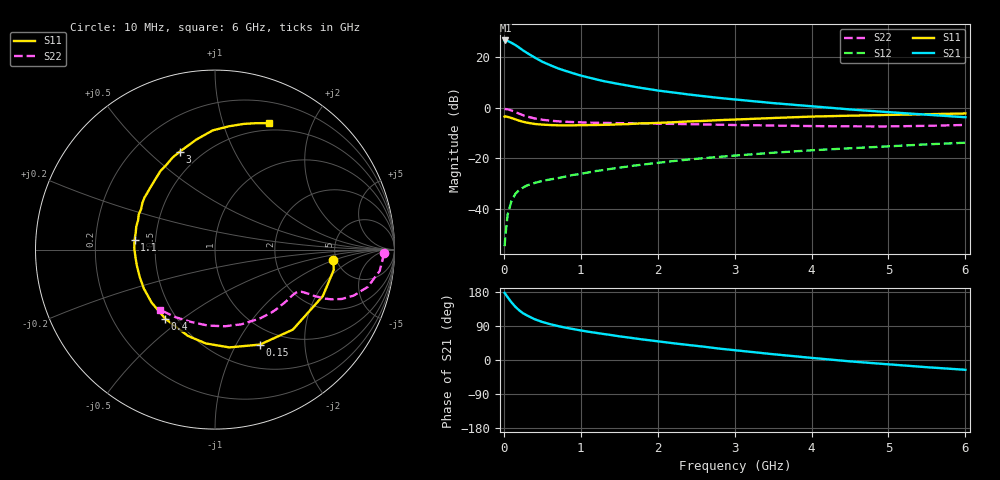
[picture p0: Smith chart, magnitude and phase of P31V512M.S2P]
! SIEMENS Small Signal Semiconductors
! BFP181
! Si NPN RF Bipolar Junction Transistor in SOT143
! VCE = 1.5 V  IC = 12 mA
! Common Emitter S-Parameters:  March  1996
# GHz  S  MA  R  50
!  f  S11  S21  S12  S22
! GHz  MAG  ANG  MAG  ANG  MAG  ANG  MAG  ANG
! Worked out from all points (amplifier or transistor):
!   36 points, 10 MHz to 6 GHz, reference 50 ohm
!   highest |S21| = 26.6 dB at 20 MHz (marker M1)
!   |S21| within 3 dB of that: start of sweep to 207.2 MHz
!   unconditionally stable (mu >= 1): 602.2 MHz to end of sweep
!   at 250 MHz: K = 0.53, MSG = 27.2 dB, |S12| = -31.7 dB
!   at 1.4 GHz: K = 1.42, MAG = 13.2 dB, |S12| = -24.2 dB
!   at 6 GHz: K = 1.16, MAG = 2.7 dB, |S12| = -13.9 dB
!   S11 on the Smith chart (normalised r, x): 10 MHz: 4.72, -0.95; 150 MHz: 0.78, -1.26; 400 MHz: 0.44, -0.43; 1.1 GHz: 0.38, +0.05; 3 GHz: 0.38, +0.63; 6 GHz: 0.42, +1.43
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0.01  0.6622 -4.9  21.39 177.0  0.0018 76.6  0.9419 -1.3
0.02  0.6712 -9.7  21.4 174.4  0.0029 80.6  0.9371 -2.9
0.05  0.6544 -23.3  20.9 165.4  0.0077 81.1  0.9252 -7.4
0.1  0.622 -45.8  19.18 151.9  0.0143 68.8  0.8765 -13.7
0.15  0.5854 -64.7  17.35 140.4  0.0196 61.8  0.8149 -18.3
0.2  0.5507 -81.7  15.42 131.1  0.0233 56.6  0.7576 -21.3
0.25  0.5252 -95.6  13.6 123.4  0.0261 52.7  0.7068 -23.1
0.3  0.5039 -107.4  12.15 117.7  0.0287 51.1  0.667 -24.1
0.4  0.4742 -125.9  9.838 107.7  0.0322 48.5  0.6109 -25.0
0.5  0.4602 -140.2  8.111 100.4  0.0352 46.5  0.5749 -25.3
0.6  0.452 -151.4  6.958 94.7  0.0377 47.5  0.5515 -25.7
0.7  0.4463 -160.0  6.021 89.8  0.04 47.7  0.5357 -26.0
0.9  0.4452 -174.5  4.799 81.7  0.0464 48.7  0.5172 -27.3
1.1  0.4512 173.0  3.955 74.6  0.0521 49.9  0.5057 -29.1
1.5  0.4676 155.4  2.927 62.5  0.0648 50.7  0.4922 -34.0
1.8  0.4884 143.6  2.436 54.3  0.074 50.3  0.4851 -38.5
2.2  0.5129 130.6  1.996 44.3  0.0871 48.6  0.4755 -45.0
3  0.5798 109.8  1.453 25.9  0.1121 44.1  0.4521 -59.9
3.5  0.6223 99.5  1.229 15.3  0.1277 40.8  0.4413 -70.6
4.5  0.6919 83.4  0.921 -3.6  0.1565 33.0  0.4253 -95.1
5.5  0.7393 72.3  0.724 -19.0  0.1873 25.4  0.4359 -120.1
6  0.7661 66.9  0.645 -25.9  0.2017 21.0  0.4538 -132.4
